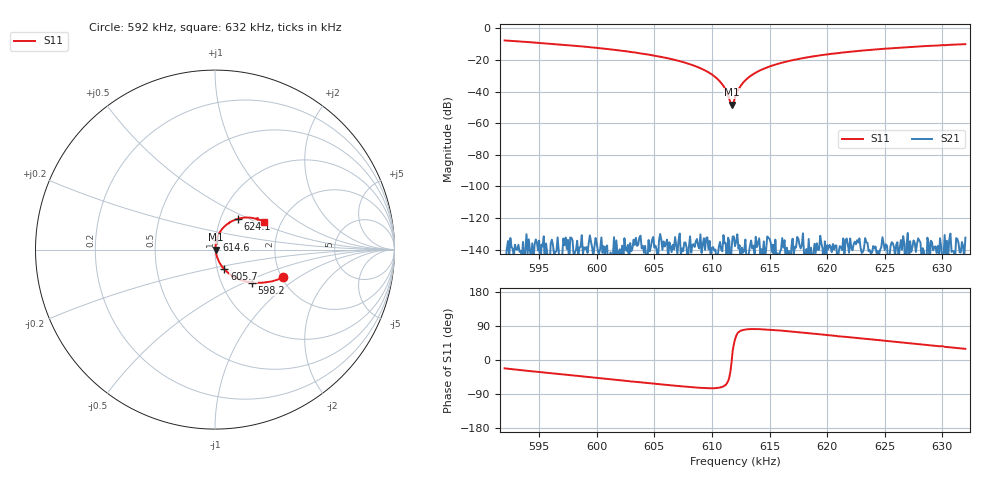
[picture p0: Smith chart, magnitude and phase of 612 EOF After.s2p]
# Hz S DB R 50
! CMT, PLANAR-814/1, 15065524, 18.3.1/3
! Date: 22/04/2020 3:15:58 AM
! Data: Format (Calibration Info)
! Freq  S11: dB/Ang (F1)  S21: dB/Ang  S12: dB/Ang  S22: dB/Ang
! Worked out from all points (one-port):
!   401 points, 592 kHz to 632 kHz, reference 50 ohm
!   lowest |S11| = -48.3 dB at 611.7 kHz (marker M1), VSWR 1.01, Z = 50.4 - j0.0437 ohm
!   |S11| at or under -10 dB: 596.3 kHz to end of sweep
!   S11 on the Smith chart (normalised r, x): 592 kHz: 2.04, -0.76; 598.2 kHz: 1.39, -0.55; 605.7 kHz: 1.08, -0.24; 614.6 kHz: 1.01, +0.11; 624.1 kHz: 1.20, +0.43; 632 kHz: 1.64, +0.56
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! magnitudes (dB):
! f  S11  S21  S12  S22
! 592 kHz  -7.7  -150.3  -  -
! 598.2 kHz  -11.2  -140.0  -  -
! 598.7 kHz  -11.5  -130.8  -  -
! 605.4 kHz  -17.9  -134.5  -  -
! 605.7 kHz  -18.3  -140.0  -  -
! 608.2 kHz  -23.0  -141.8  -  -
! 609.9 kHz  -28.8  -145.7  -  -
! 610.5 kHz  -32.2  -143.9  -  -
! 610.9 kHz  -35.5  -141.0  -  -
! 611.6 kHz  -46.8  -159.6  -  -
! 611.7 kHz  -48.3  -139.1  -  -
! 611.9 kHz  -46.5  -131.6  -  -
! 612 kHz  -43.6  -137.7  -  -
! 612.4 kHz  -37.5  -137.1  -  -
! 612.9 kHz  -32.9  -133.5  -  -
! 613.6 kHz  -28.9  -137.3  -  -
! 614.6 kHz  -25.3  -146.5  -  -
! 616.4 kHz  -21.2  -146.7  -  -
! 618.7 kHz  -17.9  -148.6  -  -
! 624.1 kHz  -13.5  -139.2  -  -
! 625.4 kHz  -12.7  -145.0  -  -
! 632 kHz  -10.1  -132.3  -  -
